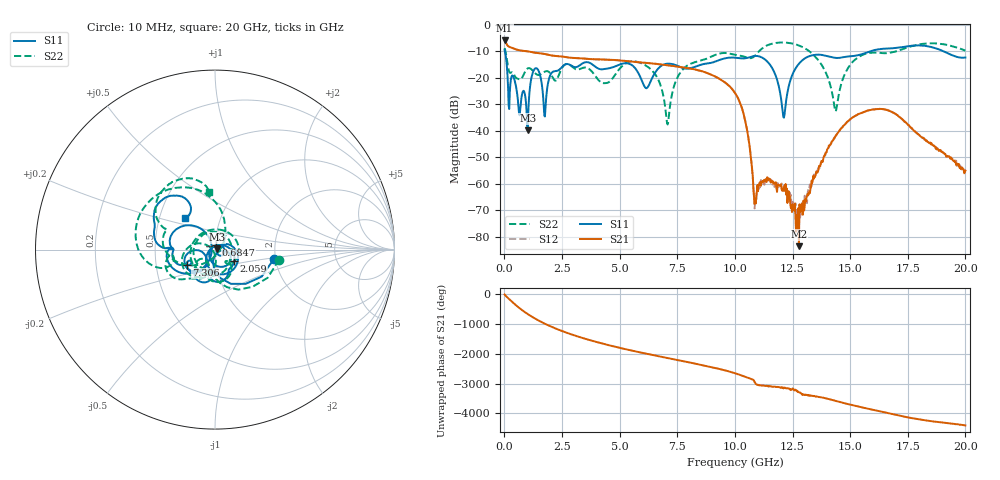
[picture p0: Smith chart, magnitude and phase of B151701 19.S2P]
!  2-Port S-parameters saved by WinCal
! VAR MeasName=S-Parameters (CALIBRATED_DATA) read from VNA (N5244A)
! VAR MeasDate=2015-12-24 19:10:23
! VAR NAME=B151701 19
! VAR FILENAME=B151701 19.S2P
! VAR DATE=2015-12-24 19:10:23
! VAR PHYS_PORTS=1,3
# Hz S DB R 50
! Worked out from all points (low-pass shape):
!   801 points, 10 MHz to 20 GHz, reference 50 ohm
!   highest |S21| = -5.95 dB at 10 MHz (marker M1); lowest = -83.6 dB at 12.78 GHz (marker M2)
!   |S21| within 3 dB of the highest: start of sweep to 387.6 MHz
!   lowest |S11| = -39.8 dB at 1.01 GHz (marker M3), VSWR 1.02, Z = 51 + j0.171 ohm
!   |S11| at or under -10 dB: 22.05 MHz to 15.89 GHz (15.87 GHz wide, 199 % of centre); 19.04 GHz to end of sweep
!   |S22| runs from -37.7 to -6.7 dB; largest |S21 - S12| = 0.00098
!   S11 on the Smith chart (normalised r, x): 10 MHz: 1.96, -0.23; 684.7 MHz: 1.01, +0.05; 2.059 GHz: 1.23, -0.16; 7.306 GHz: 0.72, -0.13; 20 GHz: 0.68, +0.25
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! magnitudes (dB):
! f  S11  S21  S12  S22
! 10 MHz  -9.6  -6.0  -6.0  -8.8
! 684.7 MHz  -32.3  -9.7  -9.7  -20.6
! 1.01 GHz  -39.8  -10.1  -10.1  -16.5
! 1.309 GHz  -16.7  -10.5  -10.5  -18.1
! 1.759 GHz  -34.6  -11.1  -11.1  -17.7
! 2.059 GHz  -18.1  -11.6  -11.6  -19.3
! 3.358 GHz  -14.8  -12.7  -12.7  -16.4
! 6.157 GHz  -24.0  -14.4  -14.4  -15.5
! 6.682 GHz  -16.5  -14.9  -14.9  -20.8
! 7.056 GHz  -14.7  -15.3  -15.3  -37.1
! 7.306 GHz  -14.9  -15.6  -15.6  -24.9
! 10.01 GHz  -12.4  -25.7  -25.7  -11.4
! 10.48 GHz  -12.7  -37.6  -37.5  -12.3
! 10.88 GHz  -11.8  -66.6  -67.2  -11.6
! 11.63 GHz  -16.5  -59.0  -60.4  -7.1
! 12.13 GHz  -35.1  -62.7  -62.8  -6.7
! 12.78 GHz  -14.7  -83.6  -72.7  -7.9
! 13.35 GHz  -11.5  -59.7  -59.2  -11.0
! 14.38 GHz  -12.5  -41.9  -41.8  -32.7
! 15.13 GHz  -11.8  -34.9  -35.0  -13.9
! 16.68 GHz  -8.9  -32.4  -32.4  -10.7
! 20 GHz  -12.4  -55.0  -55.1  -9.8
